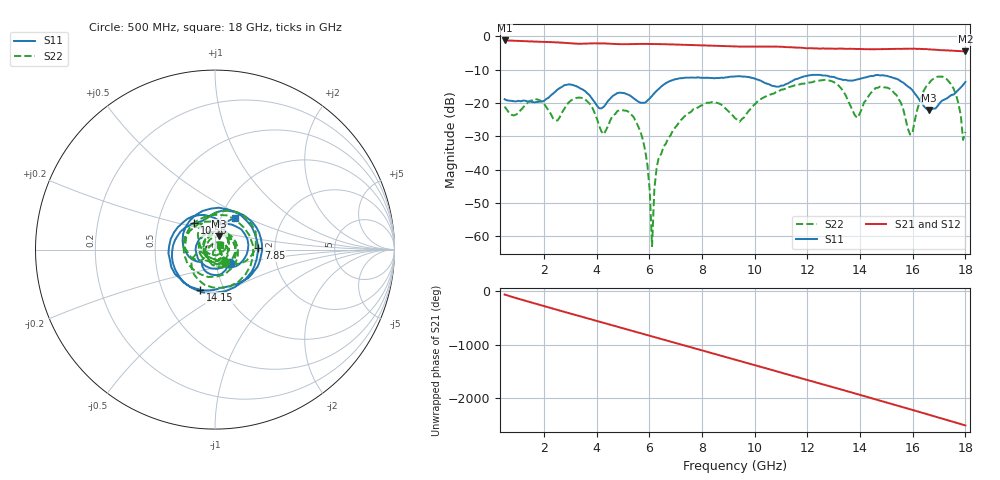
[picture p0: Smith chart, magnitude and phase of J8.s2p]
!Agilent Technologies,N5230A,MY45001360,A.07.50.67
!Agilent N5230A: A.07.50.67
!Date: Tuesday, April 16, 2024 16:03:50
!Correction: S11(Full 2 Port(1,2))
!S21(Full 2 Port(1,2))
!S12(Full 2 Port(1,2))
!S22(Full 2 Port(1,2))
!S2P File: Measurements: S11, S21, S12, S22:
# Hz S  dB  R 50
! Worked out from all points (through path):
!   201 points, 500 MHz to 18 GHz, reference 50 ohm
!   highest |S21| = -1.27 dB at 500 MHz (marker M1); lowest = -4.6 dB at 18 GHz (marker M2)
!   group delay of S21, straight-line fit = 386 ps
!   lowest |S11| = -22.2 dB at 16.6 GHz (marker M3), VSWR 1.17, Z = 51.8 + j7.75 ohm
!   |S11| at or under -10 dB: start of sweep to end of sweep
!   |S22| runs from -63.0 to -12.1 dB; largest |S21 - S12| = 0.0076
!   S11 on the Smith chart (normalised r, x): 500 MHz: 1.17, -0.18; 7.85 GHz: 1.64, +0.03; 10.56 GHz: 0.76, +0.23; 14.15 GHz: 0.77, -0.37; 18 GHz: 1.16, +0.42
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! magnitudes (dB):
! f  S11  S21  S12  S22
! 500 MHz  -18.9  -1.3  -1.3  -21.1
! 2.513 GHz  -16.0  -1.9  -1.9  -25.3
! 3.475 GHz  -16.0  -2.2  -2.2  -18.6
! 4.263 GHz  -21.2  -2.2  -2.1  -29.4
! 4.787 GHz  -17.0  -2.4  -2.4  -22.4
! 5.575 GHz  -19.6  -2.3  -2.3  -27.0
! 5.925 GHz  -19.3  -2.3  -2.3  -38.7
! 6.1 GHz  -17.9  -2.3  -2.3  -63.0
! 6.188 GHz  -17.1  -2.3  -2.3  -45.8
! 6.362 GHz  -15.8  -2.4  -2.3  -36.2
! 7.85 GHz  -12.3  -2.7  -2.7  -21.3
! 9.25 GHz  -12.1  -3.1  -3.1  -24.6
! 10.56 GHz  -14.5  -3.1  -3.1  -17.6
! 12.22 GHz  -11.6  -3.6  -3.6  -13.7
! 13.19 GHz  -12.8  -3.7  -3.7  -14.8
! 13.89 GHz  -13.0  -3.8  -3.8  -24.5
! 14.15 GHz  -12.5  -3.9  -3.9  -19.9
! 15.11 GHz  -12.1  -3.8  -3.8  -15.7
! 15.9 GHz  -15.5  -3.7  -3.8  -29.5
! 16.6 GHz  -22.2  -3.9  -4.0  -14.4
! 17.48 GHz  -17.6  -4.3  -4.2  -14.6
! 18 GHz  -13.7  -4.6  -4.6  -28.7
